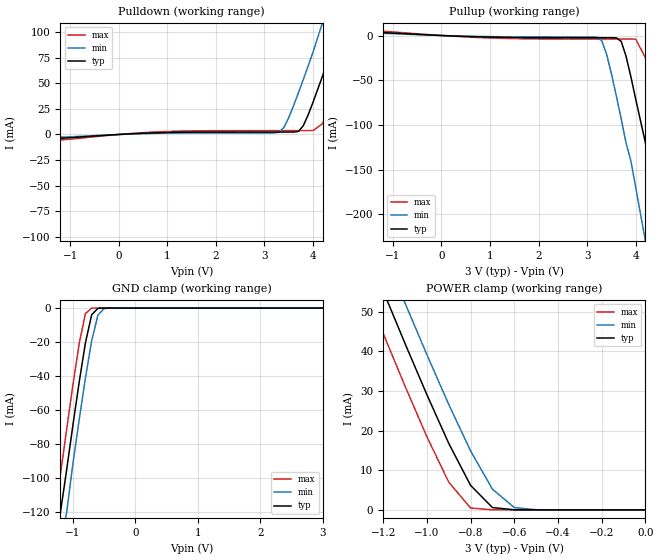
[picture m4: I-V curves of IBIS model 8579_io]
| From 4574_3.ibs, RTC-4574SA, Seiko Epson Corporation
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|   Model   8579_io
[Model] 8579_io
Model_type   I/O
Polarity   Inverting
Vinl = 0.60V
Vinh = 2.40V
C_comp   8.00pF   8.00pF   8.00pF
[Temperature Range]   25   85   -40
[Voltage Range]   3.00V   2.70V   3.30V
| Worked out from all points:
|   slope of the pulldown table from 0 to 0.45 V, typ, clamps not added: 417 ohm
|   slope of the pullup table from 0 to 0.45 V, typ, clamps not added: 474 ohm
|   GND clamp passes 1 mA (typ) near -0.62 V on its own axis
|   POWER clamp passes 1 mA (typ) near -0.71 V on its own axis
[Pulldown]
|   voltage   I(typ)   I(min)   I(max)
-3V       0A         0A         0A
-1.8V     0A         -10mA      0A
-1.6V     -5mA       -3.4mA     0A
-1.4V     -4.22mA    -3.03mA    -100mA
-1.2V     -3.71mA    -2.68mA    -5.42mA
3.3V      2.39mA     2.14mA     3.76mA
3.7V      2.97mA     40.75mA    3.76mA
4V        31.47mA    80.53mA    3.77mA
4.2V      57.68mA    110mA      10.76mA
4.6V      120mA      160mA      58.06mA
5V        170mA      220mA      110mA
6V        310mA      360mA      250mA
[Pullup]
|   voltage   I(typ)   I(min)   I(max)
-3V       0A         0A         0A
-1.2V     3.25mA     2.41mA     4.73mA
3.2V      -2.48mA    -1.88mA    -3.96mA
3.4V      -2.48mA    -20.89mA   -3.97mA
3.7V      -6.45mA    -92.89mA   -3.98mA
4V        -71.24mA   -170mA     -4.04mA
4.2V      -120mA     -230mA     -24.92mA
4.4V      -180mA     -280mA     -75.06mA
4.6V      -240mA     -340mA     -120mA
4.8V      -290mA     -390mA     -180mA
5V        -340mA     -450mA     -240mA
6V        -620mA     -740mA     -520mA
[GND_clamp]
| voltage   I(typ)   I(min)   I(max)
-3V       -620mA     -650mA     -600mA
-1.3V     -150mA     -170mA     -120mA
-1.2V     -120mA     -140mA     -97.79mA
-1.1V     -94.94mA   -120mA     -71.05mA
-1V       -68.74mA   -91.25mA   -45.09mA
-900mV    -43.52mA   -65.59mA   -20.92mA
-800mV    -20.48mA   -41.13mA   -3.17mA
-700mV    -3.96mA    -19.25mA   -37.79uA
-600mV    -140uA     -4.17mA    -260nA
-500mV    -2.83uA    -250uA     -1.81nA
3V        3.01pA     40.2nA     2.7pA
[POWER_clamp]
| voltage   I(typ)   I(min)   I(max)
-3V       310mA      320mA      300mA
-1.3V     68.77mA    78.97mA    58.06mA
-1.2V     55.29mA    65.5mA     44.54mA
-1.1V     42mA       52.22mA    31.24mA
-1V       29.08mA    39.19mA    18.48mA
-900mV    16.79mA    26.62mA    6.99mA
-800mV    6.18mA     14.88mA    470uA
-700mV    580uA      5.22mA     3.8uA
-600mV    13.83uA    580uA      26.22nA
-500mV    280nA      26.05uA    180pA
0V        3.01pA     26.81pA    3.3pA
[Ramp]
|variable   typ   min   max
dV/dt_r   0.71/1.41n   0.47/1.64n   1.05/0.97n
dV/dt_f   0.70/1.45n   0.46/1.60n   1.07/1.12n
R_load = 0.50k
|End   [Model] 8579_io
